PROGRAM MAIN_CM

VAR CONSTANT
	cInitSpectrum1 	: ST_CM_MagnitudeSpectrum_InitPars := (	nFFT_Length 		:= cFFTLength, 
															nWindowLength 		:= cWindowLength, 
															eWindowType 		:= cWindowType1,			// Hann window
															aWindowParameters	:= cWindowParameters1,
															nOverlap			:= cOverlap1,				// explicit, 50%
															eScalingType		:= cScalingType,
															bTransformToDecibel := FALSE);

	cInitSpectrum2 	: ST_CM_MagnitudeSpectrum_InitPars := (	nFFT_Length 		:= cFFTLength, 
															nWindowLength 		:= cWindowLength, 
															eWindowType 		:= cWindowType2,			// rectangular window
															aWindowParameters	:= cWindowParameters2,
															nOverlap			:= cCM_OverlapInactive,		// inactive
															eScalingType		:= cScalingType,
															bTransformToDecibel := FALSE);
															
	cInitSpectrum3 	: ST_CM_MagnitudeSpectrum_InitPars := (	nFFT_Length 		:= cFFTLength, 
															nWindowLength 		:= cWindowLength, 
															eWindowType 		:= cWindowType3,			// Bartlett window
															aWindowParameters	:= cWindowParameters3,
															nOverlap			:= cOverlap3,				// explicit, 50%
															eScalingType		:= cScalingType,
															bTransformToDecibel := FALSE);

	cInitSpectrum4 	: ST_CM_MagnitudeSpectrum_InitPars := (	nFFT_Length 		:= cFFTLength, 
															nWindowLength 		:= cWindowLength, 
															eWindowType 		:= cWindowType4,			// Hamming window
															aWindowParameters	:= cWindowParameters4,
															nOverlap			:= cOverlap4,				// explicit, 50%
															eScalingType		:= cScalingType,
															bTransformToDecibel := FALSE);
															
	cInitSpectrum5 	: ST_CM_MagnitudeSpectrum_InitPars := (	nFFT_Length 		:= cFFTLength, 
															nWindowLength 		:= cWindowLength, 
															eWindowType 		:= cWindowType5,			// Kaiser-4 window
															aWindowParameters	:= cWindowParameters5,
															nOverlap			:= cCM_OverlapRecommended,	// recommended, 67%
															eScalingType		:= cScalingType,
															bTransformToDecibel := FALSE);
															
	cInitSpectrum6 	: ST_CM_MagnitudeSpectrum_InitPars := (	nFFT_Length 		:= cFFTLength, 
															nWindowLength 		:= cWindowLength, 
															eWindowType 		:= cWindowType6,			// SFT5M FlatTop window
															aWindowParameters	:= cWindowParameters6,
															nOverlap			:= cOverlap6,				// recommended, 76%
															eScalingType		:= cScalingType,
															bTransformToDecibel := FALSE);
END_VAR

VAR	
	bCalculateOverlap	: BOOL := TRUE;
	nOverlap1			: UDINT;
	nOverlap2			: UDINT;
	nOverlap3			: UDINT;
	nOverlap4			: UDINT;
	nOverlap5			: UDINT;
	nOverlap6			: UDINT;
	
	fbSpectrum1			: FB_CMA_MagnitudeSpectrum :=(stInitPars := cInitSpectrum1, nOwnID := eID_Spectrum1, aDestIDs := [eID_Sink1]);
	fbSpectrum2			: FB_CMA_MagnitudeSpectrum :=(stInitPars := cInitSpectrum2, nOwnID := eID_Spectrum2, aDestIDs := [eID_Sink2]);
	fbSpectrum3			: FB_CMA_MagnitudeSpectrum :=(stInitPars := cInitSpectrum3, nOwnID := eID_Spectrum3, aDestIDs := [eID_Sink3]);
	fbSpectrum4			: FB_CMA_MagnitudeSpectrum :=(stInitPars := cInitSpectrum4, nOwnID := eID_Spectrum4, aDestIDs := [eID_Sink4]);
	fbSpectrum5			: FB_CMA_MagnitudeSpectrum :=(stInitPars := cInitSpectrum5, nOwnID := eID_Spectrum5, aDestIDs := [eID_Sink5]);
	fbSpectrum6			: FB_CMA_MagnitudeSpectrum :=(stInitPars := cInitSpectrum6, nOwnID := eID_Spectrum6, aDestIDs := [eID_Sink6]);
	
	// Calculate window
	bCalculateWindow	: BOOL := TRUE;
	aWindow				: ARRAY [1..cWindowLength] OF LREAL;
	aFFT				: ARRAY [1..cFFTLength/2+1] OF LREAL;
	
	// Calculate spectral scaling factors
	bCalculateFactors	: BOOL := TRUE;
	fDC_Scaling			: LREAL;
	fNonDC_Scaling		: LREAL;
	fNyquist_Scaling	: LREAL;
	
	// error monitoring
	fbErrHist			: FB_HRErrHist; 
	hr					: HRESULT;
	i					: UDINT;
END_VAR

(* Calculate overlap *)

IF bCalculateOverlap THEN
	// recommended overlap for window 1
	nOverlap1 := F_CM_CalculateRecommendedOverlap(eWindowType := cWindowType1, aWindowParameters := cWindowParameters1, nWindowLength := cWindowLength);
	
	// recommended overlap for window 2
	nOverlap2 := F_CM_CalculateRecommendedOverlap(eWindowType := cWindowType2, aWindowParameters := cWindowParameters2, nWindowLength := cWindowLength);
	
	// recommended overlap for window 3
	nOverlap3 := F_CM_CalculateRecommendedOverlap(eWindowType := cWindowType3, aWindowParameters := cWindowParameters3, nWindowLength := cWindowLength);
	
	// recommended overlap for window 4
	nOverlap4 := F_CM_CalculateRecommendedOverlap(eWindowType := cWindowType4, aWindowParameters := cWindowParameters4, nWindowLength := cWindowLength);
	
	// recommended overlap for window 5
	nOverlap5 := F_CM_CalculateRecommendedOverlap(eWindowType := cWindowType5, aWindowParameters := cWindowParameters5, nWindowLength := cWindowLength);
	
	// recommended overlap for window 6
	nOverlap6 := F_CM_CalculateRecommendedOverlap(eWindowType := cWindowType6, aWindowParameters := cWindowParameters6, nWindowLength := cWindowLength);
	
	bCalculateOverlap := FALSE;
END_IF

(* Compute spectrum *)

// Window 1
fbSpectrum1.Call();
IF fbSpectrum1.bError THEN
	fbErrHist.AddError(bErr:=TRUE, hrErrCode:=fbSpectrum1.hrErrorCode, sErrSource:='MAIN_CM.fbSpectrum1'); // error monitoring
	// ToDo: if error
END_IF

// Window 2
fbSpectrum2.Call();
IF fbSpectrum2.bError THEN
	fbErrHist.AddError(bErr:=TRUE, hrErrCode:=fbSpectrum2.hrErrorCode, sErrSource:='MAIN_CM.fbSpectrum2'); // error monitoring
	// ToDo: if error
END_IF

// Window 3
fbSpectrum3.Call();
IF fbSpectrum3.bError THEN
	fbErrHist.AddError(bErr:=TRUE, hrErrCode:=fbSpectrum3.hrErrorCode, sErrSource:='MAIN_CM.fbSpectrum3'); // error monitoring
	// ToDo: if error
END_IF

// Window 4
fbSpectrum4.Call();
IF fbSpectrum4.bError THEN
	fbErrHist.AddError(bErr:=TRUE, hrErrCode:=fbSpectrum4.hrErrorCode, sErrSource:='MAIN_CM.fbSpectrum4'); // error monitoring
	// ToDo: if error
END_IF

// Window 5
fbSpectrum5.Call();
IF fbSpectrum5.bError THEN
	fbErrHist.AddError(bErr:=TRUE, hrErrCode:=fbSpectrum5.hrErrorCode, sErrSource:='MAIN_CM.fbSpectrum5'); // error monitoring
	// ToDo: if error
END_IF

// Window 6
fbSpectrum6.Call();
IF fbSpectrum6.bError THEN
	fbErrHist.AddError(bErr:=TRUE, hrErrCode:=fbSpectrum6.hrErrorCode, sErrSource:='MAIN_CM.fbSpectrum6'); // error monitoring
	// ToDo: if error
END_IF

// Window Function
IF bCalculateWindow THEN
	hr := F_CM_CalculateWindow(cWindowType6, cWindowParameters6, cWindowLength, ADR(aWindow));
	IF SUCCEEDED(hr) THEN
		bCalculateWindow := FALSE;
	END_IF
END_IF

// Spectral scaling factors
IF bCalculateFactors THEN
	FOR i := 1 TO cFFTLength/2+1 DO
		aFFT[i] := 1.0;
	END_FOR
	hr := F_CM_ApplySpectralScaling(cScalingType, cFFTLength, 1, cSamplerate, FALSE, 2.3E-308, cWindowLength, ADR(aWindow), cFFTLength/2+1, ADR(aFFT));
	IF SUCCEEDED(hr) THEN
		bCalculateFactors := FALSE;
	END_IF
END_IF

END_PROGRAM
